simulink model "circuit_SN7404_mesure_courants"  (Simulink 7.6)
settings: Solver=ode15s  StartTime=0.0  StopTime=10  RelTol=1e-3
StopFcn:
  | clc
libraries: elec_lib x11, fl_lib x7, nesl_utility x5

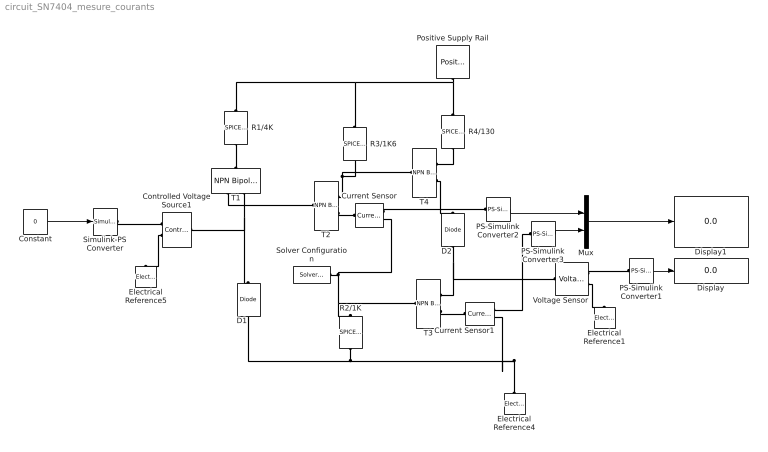
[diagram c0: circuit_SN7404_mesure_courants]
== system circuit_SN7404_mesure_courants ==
  Constant : Constant  Value=0
  Controlled Voltage Source1 : fl_lib/Electrical/Electrical Sources/Controlled Voltage Source  DialogController=NetworkEngine.DynNeDlgSource  SystemSampleTime=-1  i_Log=off  v_Log=off  LocalVarNames=|current|voltage|power  LocalVarDescs=|Current (A)|Voltage (V)|Power (W)  LocalVarLogging=[0 0 0]
  Current Sensor : fl_lib/Electrical/Electrical Sensors/Current Sensor  DialogController=NetworkEngine.DynNeDlgSource  SystemSampleTime=-1  i1_Log=off  v1_Log=off  LocalVarNames=|i1|v1  LocalVarDescs=|i1|v1  LocalVarLogging=[0 0]
  Current Sensor1 : fl_lib/Electrical/Electrical Sensors/Current Sensor  DialogController=NetworkEngine.DynNeDlgSource  SystemSampleTime=-1  i1_Log=off  v1_Log=off  LocalVarNames=|i1|v1  LocalVarDescs=|i1|v1  LocalVarLogging=[0 0]
  D1 : elec_lib/Semiconductor Devices/Diode  DialogController=NetworkEngine.DynNeDlgSource  SystemSampleTime=-1  ModelType=1  Vf=0.6 V  Ron=0.3 Ohm  Goff=1e-08 S  Rz=0.3 Ohm  Vz=50 V  C_PWL=5 pF  prmExp=1  I12="[  0.07 1.5 ] A"  V12="[  0.7 0.8 ] V"  I1=0.07 A  V1=0.7 V  RS=0.01 Ohm  IS=1e-14 A  Tmeas=25 C  ec=1  BV=Inf V  C_param=1  CJ0=5 pF  VJ=1 V  Mgrad=0.5  Vvec="[  0.1 10 100 ] V"  Cvec="[  3.5 1 0.4 ] pF"  FC=0.5  LocalVarLogging=[]
  D2 : elec_lib/Semiconductor Devices/Diode  DialogController=NetworkEngine.DynNeDlgSource  SystemSampleTime=-1  ModelType=1  Vf=0.6 V  Ron=0.3 Ohm  Goff=1e-08 S  Rz=0.3 Ohm  Vz=50 V  C_PWL=5 pF  prmExp=1  I12="[  0.07 1.5 ] A"  V12="[  0.7 0.8 ] V"  I1=0.07 A  V1=0.7 V  RS=0.01 Ohm  IS=1e-14 A  Tmeas=25 C  ec=1  BV=Inf V  C_param=1  CJ0=5 pF  VJ=1 V  Mgrad=0.5  Vvec="[  0.1 10 100 ] V"  Cvec="[  3.5 1 0.4 ] pF"  FC=0.5  LocalVarLogging=[]
  Display : Display
  Display1 : Display
  Electrical Reference1 : fl_lib/Electrical/Electrical Elements/Electrical Reference  DialogController=NetworkEngine.DynNeDlgSource  SystemSampleTime=-1  i_Log=off  LocalVarNames=|i  LocalVarDescs=|i  LocalVarLogging=[]
  Electrical Reference4 : fl_lib/Electrical/Electrical Elements/Electrical Reference  DialogController=NetworkEngine.DynNeDlgSource  SystemSampleTime=-1  i_Log=off  LocalVarNames=|i  LocalVarDescs=|i  LocalVarLogging=[]
  Electrical Reference5 : fl_lib/Electrical/Electrical Elements/Electrical Reference  DialogController=NetworkEngine.DynNeDlgSource  SystemSampleTime=-1  i_Log=off  LocalVarNames=|i  LocalVarDescs=|i  LocalVarLogging=[]
  Mux : Mux  Inputs=2
  PS-Simulink Converter1 : nesl_utility/PS-Simulink Converter  DialogController=NetworkEngine.DynNeUtilDlgSource  SystemSampleTime=-1  PhysicalDomain=network_engine_domain  LeftPortType=input  RightPortType=output  SubClassName=ps_output  Unit=V  AffineConversion=off
  PS-Simulink Converter2 : nesl_utility/PS-Simulink Converter  DialogController=NetworkEngine.DynNeUtilDlgSource  SystemSampleTime=-1  PhysicalDomain=network_engine_domain  LeftPortType=input  RightPortType=output  SubClassName=ps_output  Unit=1  AffineConversion=off
  PS-Simulink Converter3 : nesl_utility/PS-Simulink Converter  DialogController=NetworkEngine.DynNeUtilDlgSource  SystemSampleTime=-1  PhysicalDomain=network_engine_domain  LeftPortType=input  RightPortType=output  SubClassName=ps_output  Unit=A  AffineConversion=off
  Positive Supply Rail : elec_lib/Sources/Positive Supply Rail  DialogController=NetworkEngine.DynNeDlgSource  SystemSampleTime=-1  v0=5 V  current_Log=off  voltage_Log=off  power_Log=off  LocalVarNames=|current|voltage|power  LocalVarDescs=|Current (A)|Voltage (V)|Power (W)  LocalVarLogging=[0 0 0]
  R1/4K : elec_lib/Additional Components/SPICE-Compatible Components/Passive Devices/SPICE Resistor  DialogController=NetworkEngine.DynNeDlgSource  SystemSampleTime=-1  SCALE=1  R_param=1  R=4 kOhm  RSH=0 Ohm  LENGTH=1e-06 m  WIDTH=1e-06 m  NARROW=0 m  T_param=1  TC1=0 1/K  TC2=0 1/K^2  TOFFSET=0 K  TFIXED=300.15 K  TMEAS=300.15 K  LocalVarLogging=[]
  R2/1K : elec_lib/Additional Components/SPICE-Compatible Components/Passive Devices/SPICE Resistor  DialogController=NetworkEngine.DynNeDlgSource  SystemSampleTime=-1  SCALE=1  R_param=1  R=1 Ohm  RSH=0 Ohm  LENGTH=1e-06 m  WIDTH=1e-06 m  NARROW=0 m  T_param=1  TC1=0 1/K  TC2=0 1/K^2  TOFFSET=0 K  TFIXED=300.15 K  TMEAS=300.15 K  LocalVarLogging=[]
  R3/1K6 : elec_lib/Additional Components/SPICE-Compatible Components/Passive Devices/SPICE Resistor  DialogController=NetworkEngine.DynNeDlgSource  SystemSampleTime=-1  SCALE=1  R_param=1  R=1.6 kOhm  RSH=0 Ohm  LENGTH=1e-06 m  WIDTH=1e-06 m  NARROW=0 m  T_param=1  TC1=0 1/K  TC2=0 1/K^2  TOFFSET=0 K  TFIXED=300.15 K  TMEAS=300.15 K  LocalVarLogging=[]
  R4/130 : elec_lib/Additional Components/SPICE-Compatible Components/Passive Devices/SPICE Resistor  DialogController=NetworkEngine.DynNeDlgSource  SystemSampleTime=-1  SCALE=1  R_param=1  R=1.6 kOhm  RSH=0 Ohm  LENGTH=1e-06 m  WIDTH=1e-06 m  NARROW=0 m  T_param=1  TC1=0 1/K  TC2=0 1/K^2  TOFFSET=0 K  TFIXED=300.15 K  TMEAS=300.15 K  LocalVarLogging=[]
  Simulink-PS Converter : nesl_utility/Simulink-PS Converter  DialogController=NetworkEngine.DynNeUtilDlgSource  SystemSampleTime=-1  PhysicalDomain=network_engine_domain  LeftPortType=input  RightPortType=output  SubClassName=ps_input  Unit=1  AffineConversion=off  InputFilterTimeConstant=.001  UdotUserProvided=0
  Solver Configuration : nesl_utility/Solver Configuration  DialogController=NetworkEngine.DynNeUtilDlgSource  SystemSampleTime=-1  PhysicalDomain=network_engine_domain  LeftPortType=input  RightPortType=generic  SubClassName=solver  Accelerate=off  Profile=off  ResidualTolerance=1e-9  MaxNonlinIter=12  MaxModeIter=2  DoFixedCost=off  UseLocalSampling=off  DoDC=off  LinearAlgebra=Sparse  LocalSolverSampleTime=.001  LocalSolverChoice=NE_BACKWARD_EULER_ADVANCER  UseLocalSolver=off
  T{1..4} (4 alike) : elec_lib/Semiconductor Devices/NPN Bipolar Transistor  DialogController=NetworkEngine.DynNeDlgSource  SystemSampleTime=-1  parameterization=1  BF=100  IS=1e-14 A  VAF=200 V  hfe=100  hoe=5e-05 1/Ohm  Ic_h=1 mA  V1=0.55 V  I1=0.5 mA  BR=1  Tmeas=25 C  RC=0.1 Ohm  RE=0.1 Ohm  RB=0.1 Ohm  C_BC=5 pF  C_BE=5 pF  TF=0 us  TR=0 us  LocalVarLogging=[]
  Voltage Sensor : fl_lib/Electrical/Electrical Sensors/Voltage Sensor  DialogController=NetworkEngine.DynNeDlgSource  SystemSampleTime=-1  i1_Log=off  v1_Log=off  LocalVarNames=|i1|v1  LocalVarDescs=|i1|v1  LocalVarLogging=[0 0]
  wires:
  Constant/1 -> Simulink-PS Converter/1
  PS-Simulink Converter1/1 -> Display/1
  PS-Simulink Converter2/1 -> Mux/1
  PS-Simulink Converter3/1 -> Mux/2
  Mux/1 -> Display1/1
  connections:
  Voltage Sensor/RConn1 -- PS-Simulink Converter1/LConn1
  Voltage Sensor/RConn2 -- Electrical Reference1/LConn1
  R1/4K/RConn1 -- T1/LConn1
  Positive Supply Rail/RConn1 -- R1/4K/LConn1 -- R3/1K6/LConn1 -- R4/130/LConn1
  T1/RConn2 -- D1/RConn1 -- Controlled Voltage Source1/LConn1
  T1/RConn1 -- T2/LConn1
  Solver Configuration/RConn1 -- R2/1K/LConn1 -- T3/LConn1 -- Current Sensor/RConn2
  T2/RConn1 -- T4/LConn1 -- R3/1K6/RConn1
  R4/130/RConn1 -- T4/RConn1
  T4/RConn2 -- D2/LConn1
  D2/RConn1 -- T3/RConn1 -- Voltage Sensor/LConn1
  Controlled Voltage Source1/RConn2 -- Electrical Reference5/LConn1
  Simulink-PS Converter/RConn1 -- Controlled Voltage Source1/RConn1
  T2/RConn2 -- Current Sensor/LConn1
  T3/RConn2 -- Current Sensor1/LConn1
  R2/1K/RConn1 -- Current Sensor1/RConn2 -- Electrical Reference4/LConn1 -- D1/LConn1
  Current Sensor/RConn1 -- PS-Simulink Converter2/LConn1
  PS-Simulink Converter3/LConn1 -- Current Sensor1/RConn1
